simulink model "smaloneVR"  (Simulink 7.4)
settings: Solver=ode23t  StartTime=0.0  StopTime=4  MaxStep=0.01  RelTol=1e-5  AbsTol=1e-4
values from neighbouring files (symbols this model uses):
  Ef = parEf(m)    [Ccurverun.m]
  Ra = .95    (= 0.95)    [altwdgs.m]    (also in Ccurverun.m = 0.018)
  wo = 2*pi*freq0    [calc0.m]    (also in IMabc2.m = 376.991118431; imabcparam.m = 376.991118431; IMabcrun0.m = 376.991118431; IMabcrun1.m = 376.991118431)
undefined symbols (not defined in the file or in its folder): fa0, fk0, Lal, Lfl, Lkdl, Lkql, Lload, Lmd, Lmq, phif0, Rf, Rkd, Rkq, Rload, vf0

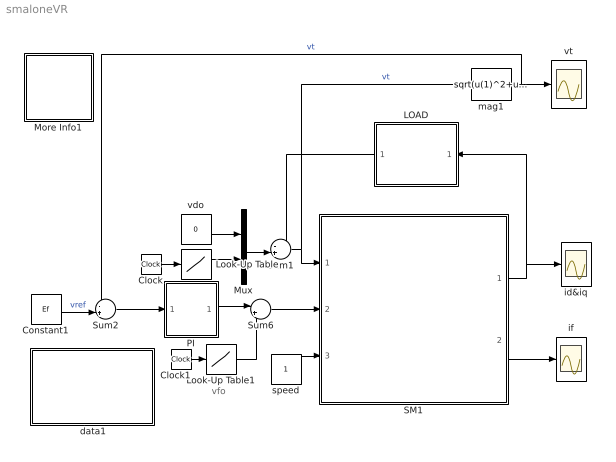
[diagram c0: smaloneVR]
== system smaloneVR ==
  note: vfo
  " data1" : Subsystem
  Clock : Clock
  Clock1 : Clock
  Constant1 : Constant  Value=Ef  OutDataType=sfix(16)  OutScaling=2^0
  LOAD : Subsystem
  Look-Up Table : Lookup  InputValues=[0 0.5 0.51 20]  Table="[Ef Ef  0 0]"  OutDataType=sfix(16)  OutScaling=2^0
  Look-Up Table1 : Lookup  InputValues=[0 0.5 0.54 20]  Table=[vf0 vf0 0 0]  OutDataType=sfix(16)  OutScaling=2^0
  More Info1 : Subsystem
  Mux : Mux  Inputs=2
  PI : Subsystem
  SM1 : Subsystem
  Sum1 : Sum  Inputs=-+|  OutDataType=sfix(16)  OutScaling=2^0
  Sum2 : Sum  Inputs=-+|  OutDataType=sfix(16)  OutScaling=2^0
  Sum6 : Sum  Inputs=|++  OutDataType=sfix(16)  OutScaling=2^0
  id&iq : Scope
  if : Scope
  mag1 : Fcn  Expr=sqrt(u(1)^2+u(2)^2)
  speed : Constant  OutDataType=sfix(16)  OutScaling=2^0
  vdo : Constant  Value=0  OutDataType=sfix(16)  OutScaling=2^0
  vt : Scope
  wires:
  SM1/2(if) -> if/1
  speed/1 -> SM1/3(wm)
  Look-Up Table/1 -> Mux/2
  Mux/1 -> Sum1/2
  LOAD/1(v_out) -> Sum1/1
  Sum1/1 -> SM1/1(vs), mag1/1  "vt"
  Clock/1 -> Look-Up Table/1
  Constant1/1 -> Sum2/2  "vref"
  Sum2/1 -> PI/1(we)
  mag1/1 -> vt/1, Sum2/1  "vt"
  vdo/1 -> Mux/1
  SM1/1(ia) -> id&iq/1, LOAD/1("i_in ")
  Clock1/1 -> Look-Up Table1/1
  Look-Up Table1/1 -> Sum6/2
  Sum6/1 -> SM1/2(vf)
  PI/1(wr) -> Sum6/1

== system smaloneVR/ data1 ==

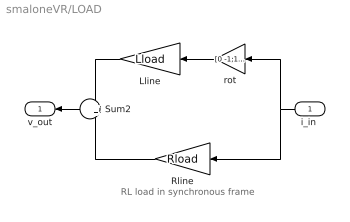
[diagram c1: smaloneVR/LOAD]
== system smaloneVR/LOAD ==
  note: RL load in synchronous frame
  "i_in " : Inport  OutDataType=sfix(16)  OutScaling=2^0
  Lline : Gain  Gain=Lload  ParameterDataType=sfix(16)  ParameterScaling=2^0  OutDataType=sfix(16)  OutScaling=2^0
  Rline : Gain  Gain=Rload  ParameterDataType=sfix(16)  ParameterScaling=2^0  OutDataType=sfix(16)  OutScaling=2^0
  Sum2 : Sum  OutDataType=sfix(16)  OutScaling=2^0
  rot : Gain  Gain=[0 -1;1 0]  Multiplication=Matrix(K*u)  ParameterDataType=sfix(16)  ParameterScaling=2^0  OutDataType=sfix(16)  OutScaling=2^0
  v_out : Outport
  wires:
  "i_in "/1 -> rot/1, Rline/1
  rot/1 -> Lline/1
  Lline/1 -> Sum2/1
  Rline/1 -> Sum2/2
  Sum2/1 -> v_out/1

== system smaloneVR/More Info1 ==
  note: The generator runs under open-cicuit conditions when an inductive-resistive load is suddenly applied. The model is simplified by assuming constant synchronous speed operation. The voltage regulator is represented by a PI controller.
  note: Synchronous generator with voltage regulator

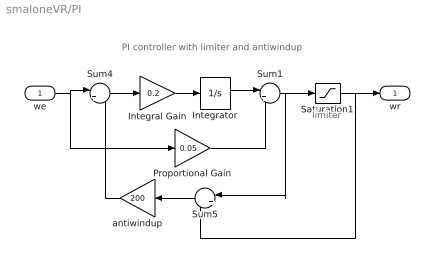
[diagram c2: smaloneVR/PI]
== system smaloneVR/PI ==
  note: PI controller with limiter and antiwindup
  note: limiter
  we : Inport  OutDataType=sfix(16)  OutScaling=2^0
  Integral Gain : Gain  Gain=0.2  ParameterDataType=sfix(16)  ParameterScaling=2^0  OutDataType=sfix(16)  OutScaling=2^0
  Integrator : Integrator
  Proportional Gain : Gain  Gain=0.05  ParameterDataType=sfix(16)  ParameterScaling=2^0  OutDataType=sfix(16)  OutScaling=2^0
  Saturation1 : Saturate  UpperLimit=.005  LowerLimit=-.005
  Sum1 : Sum  Inputs=|++  OutDataType=sfix(16)  OutScaling=2^0
  Sum4 : Sum  Inputs=|+-  OutDataType=sfix(16)  OutScaling=2^0
  Sum5 : Sum  Inputs=|+-  OutDataType=sfix(16)  OutScaling=2^0
  antiwindup : Gain  Gain=200  ParameterDataType=sfix(16)  ParameterScaling=2^0  OutDataType=sfix(16)  OutScaling=2^0
  wr : Outport
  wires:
  Saturation1/1 -> Sum5/2, wr/1
  antiwindup/1 -> Sum4/2
  Sum5/1 -> antiwindup/1
  Sum1/1 -> Sum5/1, Saturation1/1
  Sum4/1 -> Integral Gain/1
  we/1 -> Proportional Gain/1, Sum4/1
  Proportional Gain/1 -> Sum1/2
  Integrator/1 -> Sum1/1
  Integral Gain/1 -> Integrator/1

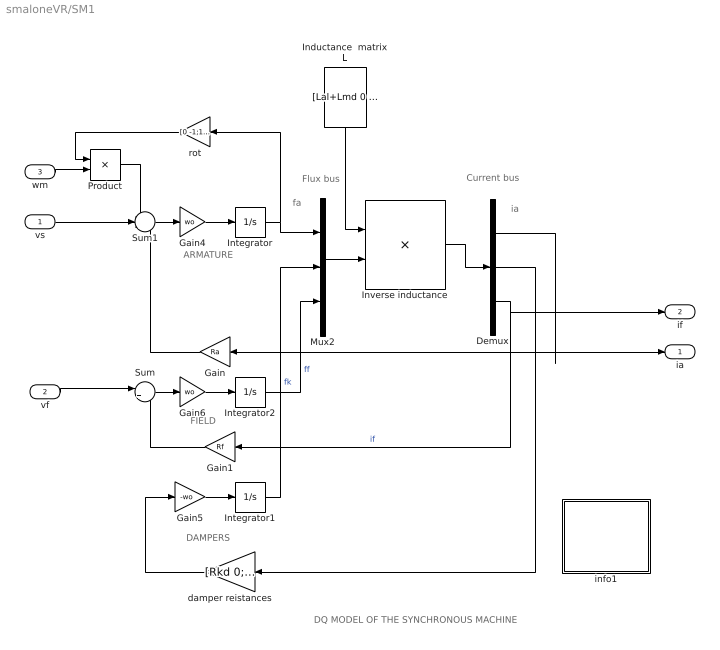
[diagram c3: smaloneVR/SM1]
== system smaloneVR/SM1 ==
  note: DAMPERS
  note: ARMATURE
  note: fa
  note: ia
  note: FIELD
  note: DQ MODEL OF THE SYNCHRONOUS MACHINE
  note: Flux bus
  note: Current bus
  vs : Inport  OutDataType=sfix(16)  OutScaling=2^0
  vf : Inport  Port=2  OutDataType=sfix(16)  OutScaling=2^0
  wm : Inport  Port=3  OutDataType=sfix(16)  OutScaling=2^0
  Demux : Demux  Outputs=3
  Gain : Gain  Gain=Ra  ParameterDataType=sfix(16)  ParameterScaling=2^0  OutDataType=sfix(16)  OutScaling=2^0
  Gain1 : Gain  Gain=Rf  ParameterDataType=sfix(16)  ParameterScaling=2^0  OutDataType=sfix(16)  OutScaling=2^0
  Gain4 : Gain  Gain=wo  ParameterDataType=sfix(16)  ParameterScaling=2^0  OutDataType=sfix(16)  OutScaling=2^0
  Gain5 : Gain  Gain=-wo  ParameterDataType=sfix(16)  ParameterScaling=2^0  OutDataType=sfix(16)  OutScaling=2^0
  Gain6 : Gain  Gain=wo  ParameterDataType=sfix(16)  ParameterScaling=2^0  OutDataType=sfix(16)  OutScaling=2^0
  Inductance  matrix L : Constant  Value=[Lal+Lmd 0 Lmd 0 Lmd;0 Lal+Lmq 0 Lmq 0;Lmd 0 Lmd+Lkdl 0 Lmd;0 Lmq 0 Lmq+Lkql 0;Lmd 0 Lmd 0 Lmd+Lfl]  VectorParams1D=off  OutDataType=fixdt(1, 16)  OutScaling=2^0
  Integrator : Integrator  InitialCondition=fa0
  Integrator1 : Integrator  InitialCondition=fk0
  Integrator2 : Integrator  InitialCondition=phif0
  Inverse inductance : Product  Inputs=/*  Multiplication=Matrix(*)  OutDataType=sfix(16)  OutScaling=2^0
  Mux2 : Mux  Inputs=3
  Product : Product  OutDataType=sfix(16)  OutScaling=2^0
  Sum : Sum  Inputs=|+-  OutDataType=sfix(16)  OutScaling=2^0
  Sum1 : Sum  Inputs=-+-  OutDataType=sfix(16)  OutScaling=2^0
  damper reistances : Gain  Gain=[Rkd 0;0 Rkq]  Multiplication=Matrix(K*u)  ParameterDataType=sfix(16)  ParameterScaling=2^0  OutDataType=sfix(16)  OutScaling=2^0
  info1 : Subsystem
  rot : Gain  Gain=[0 -1;1 0]  Multiplication=Matrix(K*u)  ParameterDataType=sfix(16)  ParameterScaling=2^0  OutDataType=sfix(16)  OutScaling=2^0
  ia : Outport
  if : Outport  Port=2
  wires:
  Product/1 -> Sum1/1
  rot/1 -> Product/1
  wm/1 -> Product/2
  Gain5/1 -> Integrator1/1
  damper reistances/1 -> Gain5/1
  Integrator/1 -> Mux2/1, rot/1
  Sum1/1 -> Gain4/1
  Gain4/1 -> Integrator/1
  vs/1 -> Sum1/2
  Gain/1 -> Sum1/3
  Gain6/1 -> Integrator2/1
  Sum/1 -> Gain6/1
  vf/1 -> Sum/1
  Gain1/1 -> Sum/2
  Demux/1 -> Gain/1, ia/1
  Integrator1/1 -> Mux2/2  "fk"
  Integrator2/1 -> Mux2/3  "ff"
  Demux/2 -> damper reistances/1
  Demux/3 -> if/1, Gain1/1  "if"
  Mux2/1 -> Inverse inductance/2
  Inverse inductance/1 -> Demux/1
  Inductance  matrix L/1 -> Inverse inductance/1

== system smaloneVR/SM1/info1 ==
  note: Synchronous machine transients under shortcircuit
  note: This demonstration illustrates the dynamics of a synchronous generator, initially at no load, following a three-phase short circuit at the terminals.
